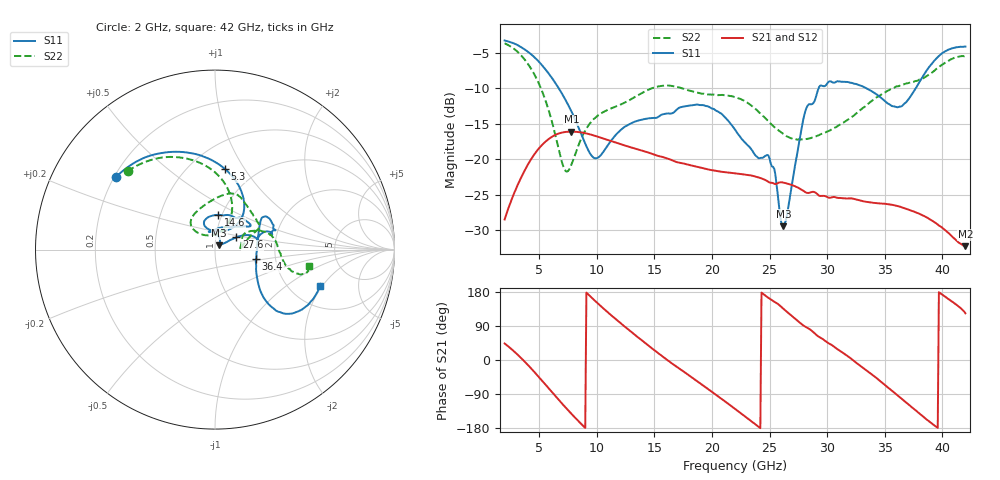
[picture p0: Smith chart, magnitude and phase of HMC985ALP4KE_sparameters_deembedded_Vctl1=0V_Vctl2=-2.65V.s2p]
!s2p File: Measurements: S11, S21, S12, S22
# GHz S dB R 50.0
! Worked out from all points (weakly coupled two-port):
!   401 points, 2 GHz to 42 GHz, reference 50 ohm
!   highest |S21| = -16.11 dB at 7.8 GHz (marker M1); lowest = -32.2 dB at 42 GHz (marker M2)
!   lowest |S11| = -29.4 dB at 26.2 GHz (marker M3), VSWR 1.07, Z = 52.3 + j2.59 ohm
!   |S11| at or under -10 dB: 6.693 GHz to 29.26 GHz (22.57 GHz wide, 126 % of centre); 33.38 GHz to 37.7 GHz (4.316 GHz wide, 12.1 % of centre)
!   |S22| runs from -21.7 to -3.7 dB; largest |S21 - S12| = 0.00066
!   S11 on the Smith chart (normalised r, x): 2 GHz: 0.21, +0.31; 5.3 GHz: 0.73, +0.82; 14.6 GHz: 0.96, +0.39; 27.6 GHz: 1.25, +0.17; 36.4 GHz: 1.58, -0.18; 42 GHz: 2.91, -1.90
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2  -3.29 144.0  -28.46 43.7  -28.46 43.7  -3.69 138.1
3.5  -4.30 117.4  -22.35 3.1  -22.37 3.1  -5.52 107.1
5.3  -6.87 83.1  -17.90 -56.3  -17.92 -56.4  -10.62 72.0
7.1  -11.11 54.3  -16.20 -118.9  -16.23 -118.9  -21.01 82.9
7.8  -13.27 49.2  -16.11 -142.0  -16.12 -142.1  -20.76 120.1
8.7  -16.64 52.7  -16.23 -170.2  -16.22 -170.2  -16.91 136.5
10  -19.84 88.4  -16.78 151.9  -16.78 151.9  -13.96 132.7
14.6  -14.22 84.4  -19.12 35.3  -19.09 35.3  -10.14 79.9
15.4  -13.97 73.7  -19.56 16.7  -19.57 16.7  -9.73 73.6
19.3  -12.41 33.9  -21.28 -68.7  -21.29 -68.7  -10.78 43.5
22  -15.82 52.2  -21.97 -128.8  -22.01 -128.8  -11.26 26.4
25  -19.90 99.1  -23.27 162.0  -23.23 162.0  -14.84 15.8
26.2  -29.44 47.1  -23.28 135.2  -23.32 135.2  -16.46 5.4
27.6  -17.30 29.9  -24.10 99.1  -24.10 99.0  -17.19 -0.6
28.1  -13.26 21.0  -24.62 87.9  -24.66 87.8  -17.18 0.8
28.7  -12.24 13.0  -24.59 76.1  -24.60 76.1  -16.94 4.6
31  -9.05 23.3  -25.44 26.4  -25.43 26.5  -15.23 26.4
33.3  -9.93 34.2  -25.96 -24.8  -25.94 -24.8  -12.55 26.2
35.4  -12.27 11.9  -26.34 -75.2  -26.32 -75.3  -10.26 17.3
36.4  -12.58 -13.2  -26.70 -100.6  -26.74 -100.6  -9.55 11.4
39.5  -5.82 -43.4  -29.05 -176.8  -29.02 -176.8  -7.28 -14.7
42  -4.15 -18.9  -32.21 123.2  -32.20 123.4  -5.48 -9.7
